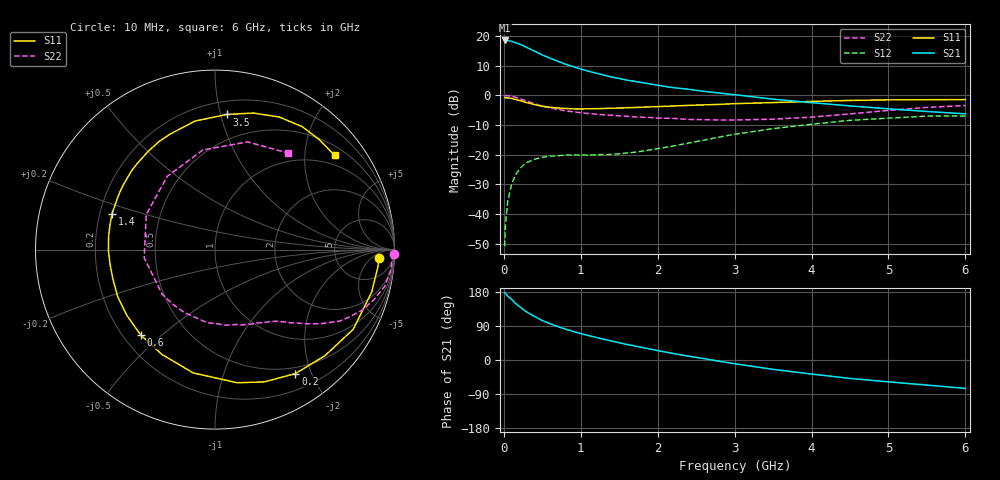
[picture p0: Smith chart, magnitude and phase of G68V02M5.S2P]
! SIEMENS Small Signal Semiconductors
! BFG193
! Si NPN RF Bipolar Junction Transistor in SOT223
! VCE = 8 V  IC = 2.5 mA
! Common Emitter S-Parameters:  August  1996
# GHz  S  MA  R  50
!  f  S11  S21  S12  S22
! GHz  MAG  ANG  MAG  ANG  MAG  ANG  MAG  ANG
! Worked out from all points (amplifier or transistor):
!   36 points, 10 MHz to 6 GHz, reference 50 ohm
!   highest |S21| = 18.5 dB at 10 MHz (marker M1)
!   |S21| within 3 dB of that: start of sweep to 350.4 MHz
!   unconditionally stable (mu >= 1): 1.332 GHz to 2.521 GHz
!   at 250 MHz: K = 0.20, MSG = 20.2 dB, |S12| = -23.6 dB
!   at 1.4 GHz: K = 1.04, MAG = 11.8 dB, |S12| = -19.9 dB
!   at 6 GHz: K = 0.92, MSG = 0.4 dB, |S12| = -6.9 dB
!   S11 on the Smith chart (normalised r, x): 10 MHz: 16, -10; 200 MHz: 0.41, -1.77; 600 MHz: 0.27, -0.43; 1.4 GHz: 0.25, +0.16; 3.5 GHz: 0.30, +1.05; 6 GHz: 0.72, +2.71
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0.01  0.9146 -3.1  8.383 177.6  0.0029 92.0  0.9961 -1.4
0.02  0.9122 -6.3  8.377 176.5  0.0063 89.7  0.9867 -2.5
0.05  0.9047 -15.1  8.355 168.8  0.0164 80.0  0.9874 -6.3
0.1  0.8892 -29.9  8.11 160.3  0.0317 74.6  0.967 -12.3
0.15  0.8516 -43.9  7.688 149.5  0.0454 65.7  0.9266 -17.7
0.2  0.8233 -57.0  7.326 141.7  0.0567 60.2  0.888 -22.2
0.25  0.7867 -69.5  6.863 133.5  0.0663 53.7  0.8391 -26.5
0.3  0.7523 -80.5  6.37 126.4  0.0743 49.0  0.8011 -29.8
0.4  0.6977 -100.0  5.536 114.8  0.0842 41.1  0.7209 -34.9
0.5  0.6548 -116.9  4.773 104.1  0.0907 34.9  0.66 -38.8
0.6  0.6303 -131.1  4.222 95.7  0.0948 30.9  0.6155 -41.7
0.8  0.6023 -154.1  3.344 81.5  0.0985 26.0  0.5506 -46.9
0.9  0.5924 -163.6  3.036 75.3  0.0992 25.1  0.5279 -49.1
1.1  0.5939 -179.5  2.55 64.6  0.0996 24.5  0.4943 -54.9
1.4  0.6077 160.8  2.033 50.1  0.1014 26.6  0.462 -63.9
1.6  0.6183 149.7  1.8 40.9  0.107 29.2  0.4443 -70.9
2.2  0.6613 124.6  1.348 17.2  0.1405 34.9  0.4096 -96.0
2.8  0.7046 104.4  1.093 -3.3  0.1987 31.2  0.385 -128.1
3.5  0.7558 85.0  0.862 -24.7  0.2754 17.4  0.3974 -173.4
4.5  0.821 64.1  0.664 -48.6  0.3801 -5.9  0.4871 123.1
5.5  0.8445 46.6  0.535 -66.2  0.4473 -34.6  0.6269 73.2
6  0.8485 38.3  0.489 -75.0  0.4511 -50.2  0.6753 52.7
